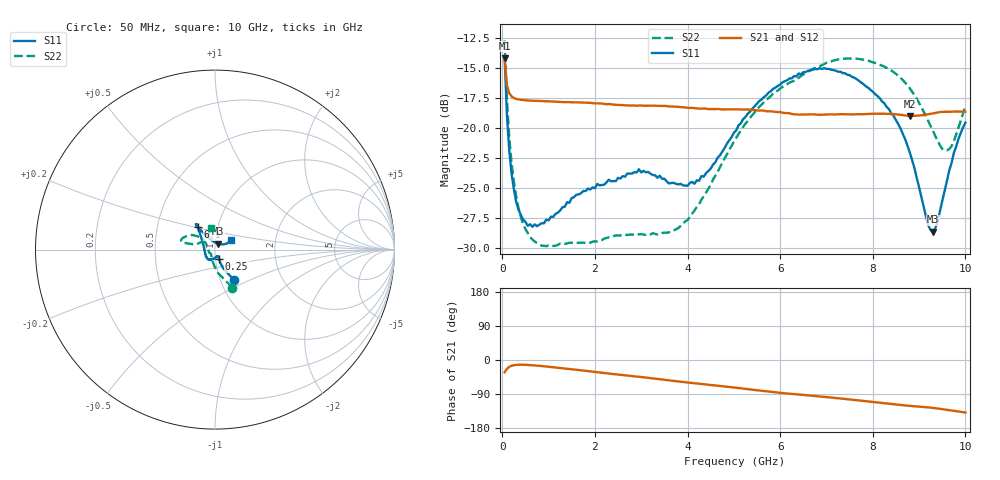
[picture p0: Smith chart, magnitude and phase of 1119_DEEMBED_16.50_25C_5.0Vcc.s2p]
!Hittite Microwave Corp.
!Digital Attenuator/PhaseShifter Rev 1.4.0
!Filename: C:\DATA\DATA\1119_DEEMBED_16.50_25C_5.0Vcc.s2p
!VNA ID: Agilent Technologies,N5224A,MY51441122,A.10.45.03
!Device type:
!2 Port Calibration.
!Temp(C): 25
!Lot Number:
!Serial Number:
!Operator:
!Misc:
!Attenuator:  16.500
# GHZ S DB R 50.0
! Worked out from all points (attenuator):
!   200 points, 50 MHz to 10 GHz, reference 50 ohm
!   highest |S21| = -14.13 dB at 50 MHz (marker M1); lowest = -19.0 dB at 8.8 GHz (marker M2)
!   lowest |S11| = -28.7 dB at 9.3 GHz (marker M3), VSWR 1.08, Z = 51.4 + j3.48 ohm
!   |S11| at or under -10 dB: start of sweep to end of sweep
!   |S22| runs from -29.9 to -12.7 dB; largest |S21 - S12| = 0.00041
!   S11 on the Smith chart (normalised r, x): 50 MHz: 1.16, -0.41; 250 MHz: 1.04, -0.11; 6.1 GHz: 0.80, +0.21; 10 GHz: 1.19, +0.13
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0.05  -14.05 -58.1  -14.13 -32.3  -14.13 -32.4  -12.67 -65.3
0.1  -18.93 -66.4  -16.43 -23.4  -16.43 -23.3  -17.62 -82.7
0.15  -21.82 -68.0  -17.09 -18.1  -17.08 -18.1  -20.75 -92.3
0.25  -25.11 -66.3  -17.48 -13.7  -17.48 -13.7  -24.48 -104.8
0.4  -27.27 -65.7  -17.63 -12.4  -17.63 -12.4  -27.45 -116.8
0.65  -28.26 -69.6  -17.71 -13.8  -17.71 -13.9  -29.32 -128.1
1.75  -25.26 -103.6  -17.87 -27.9  -17.87 -27.9  -29.59 -137.9
2.95  -23.45 -126.8  -18.11 -44.2  -18.12 -44.3  -28.89 -157.0
3.4  -23.99 -143.9  -18.14 -50.7  -18.15 -50.8  -28.84 -170.3
3.8  -24.72 -162.4  -18.22 -56.6  -18.23 -56.7  -28.37 174.0
4.15  -24.66 179.1  -18.33 -61.5  -18.34 -61.5  -26.91 159.1
5.05  -20.20 140.3  -18.43 -73.2  -18.45 -73.3  -20.83 140.5
6.1  -16.08 127.0  -18.74 -87.9  -18.76 -87.9  -16.42 147.4
6.7  -15.12 126.8  -18.85 -94.5  -18.86 -94.5  -15.06 155.0
7.5  -15.57 127.8  -18.85 -104.2  -18.86 -104.2  -14.18 164.0
8.35  -18.42 125.3  -18.82 -115.4  -18.82 -115.4  -15.07 167.5
8.8  -22.04 119.3  -18.98 -121.0  -18.98 -121.0  -16.67 167.2
9.2  -28.15 86.1  -18.84 -125.1  -18.85 -125.2  -19.44 162.8
9.3  -28.66 66.4  -18.77 -126.5  -18.79 -126.5  -20.23 158.7
9.5  -26.10 37.1  -18.65 -129.7  -18.66 -129.7  -21.74 143.2
9.65  -23.56 28.4  -18.63 -132.3  -18.64 -132.3  -21.76 126.6
10  -19.55 30.4  -18.63 -138.6  -18.64 -138.6  -18.11 99.5
